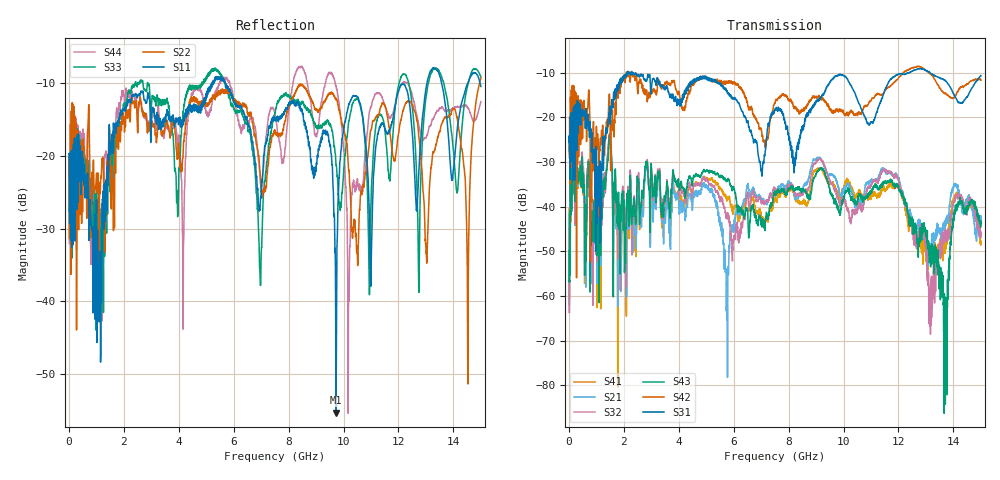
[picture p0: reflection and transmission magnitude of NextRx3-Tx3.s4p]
! FILE: N:\QM 2007\Prüfprotokolle\Highspeed\Konfektionierte Ltg\L45593-D106\D30\8216\0002\Next  Platine 2\NextRx3-Tx3.s4p
# MHz S DB R 50.00
! FREQ  S11  S12  S13  S14
!  S21  S22  S23  S24
!  S31  S32  S33  S34
!  S41  S42  S43  S44
!  DB  ANG  DB  ANG  DB  ANG  DB  ANG
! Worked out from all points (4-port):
!   2999 points, 10 MHz to 15 GHz, reference 50 ohm
!   strongest paths, dB at 10 MHz, 3.755 GHz, 7.505 GHz, 11.26 GHz, 15 GHz:
!     S31: -25.6, -15.8, -18.3, -17.9, -10.6
!     S42: -25.0, -11.7, -16.9, -14.8, -11.7
!     S43: -49.8, -35.1, -36.9, -36.0, -43.9
!     S32: -44.9, -34.8, -36.0, -34.4, -46.9
!     S21: -41.7, -38.6, -35.9, -33.6, -44.2
!     S41: -40.5, -37.7, -38.3, -37.2, -48.6
!   lowest |S11| = -55.3 dB at 9.72 GHz (marker M1), VSWR 1.00, Z = 49.9 + j0.124 ohm
!   |S11| at or under -10 dB: start of sweep to 5.212 GHz; 5.698 GHz to 13.03 GHz (7.336 GHz wide, 78.3 % of centre); 13.57 GHz to 14.52 GHz (948.7 MHz wide, 6.75 % of centre)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
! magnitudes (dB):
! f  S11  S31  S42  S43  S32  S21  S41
! 10 MHz  -19.8  -25.6  -25.0  -49.8  -44.9  -41.7  -40.5
! 8.32 GHz  -12.7  -26.8  -18.5  -36.2  -37.4  -37.0  -38.4
! 9.72 GHz  -55.3  -10.9  -18.2  -39.4  -36.1  -33.8  -36.0
! 10.2 GHz  -12.8  -12.1  -18.9  -36.3  -41.4  -35.3  -34.6
! 13.71 GHz  -13.1  -11.9  -14.6  -66.9  -46.4  -43.7  -48.7
! 14.53 GHz  -10.0  -15.2  -12.5  -40.5  -39.7  -37.8  -39.5
! 15 GHz  -10.4  -10.6  -11.7  -43.9  -46.9  -44.2  -48.6
